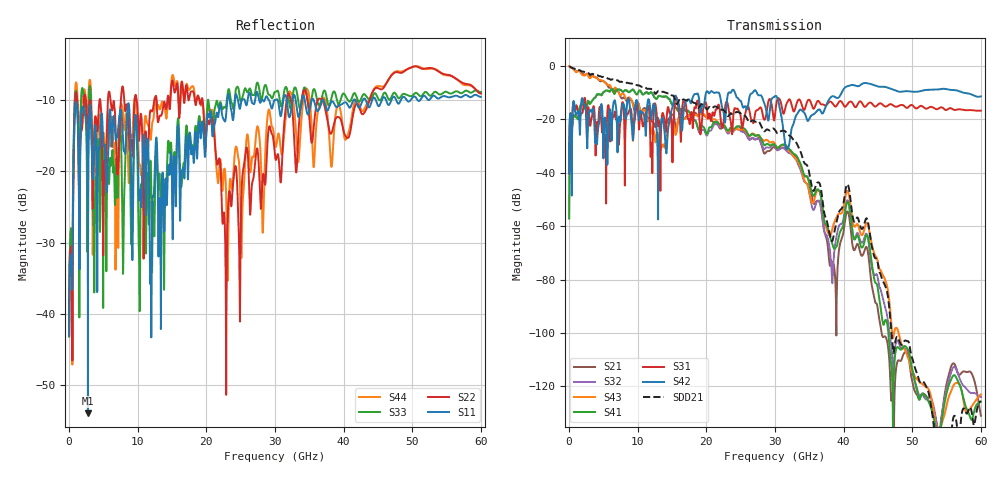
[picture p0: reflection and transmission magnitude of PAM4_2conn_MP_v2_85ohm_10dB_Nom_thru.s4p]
! Info: Touchstone file created by Circ.  Input file=FAB50GbE_2conn_Midplane_Examax_Topo2_v2_85ohm_10dB_Nom.circ
# Hz S RI R 50
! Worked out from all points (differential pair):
!   6000 points, 10 MHz to 60 GHz, reference 50 ohm
!   strongest paths, dB at 10 MHz, 15.01 GHz, 30.01 GHz, 45.01 GHz, 60 GHz:
!     S42: -40.2, -15.9, -11.3, -7.7, -11.4
!     S31: -40.3, -28.2, -18.4, -14.5, -16.7
!     S41: -57.1, -14.4, -29.7, -83.7, -125.7
!     S43: -0.1, -20.4, -29.2, -73.8, -123.0
!     S32: -57.1, -14.5, -30.1, -79.8, -124.0
!     S21: -0.1, -18.2, -30.7, -91.5, -131.0
!   taken as a pair (ports 3,1 in; 4,2 out), SDD21 dB: -0.1, -11.1, -24.0, -74.3, -125.5
!   lowest |S11| = -53.9 dB at 2.75 GHz (marker M1), VSWR 1.00, Z = 50.2 + j0.0695 ohm
!   |S11| at or under -10 dB: start of sweep to 23.06 GHz; 35.65 GHz to 36.88 GHz (1.236 GHz wide, 3.41 % of centre); 37.06 GHz to 41.45 GHz (4.386 GHz wide, 11.2 % of centre)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
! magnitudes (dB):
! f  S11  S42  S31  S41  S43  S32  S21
! 10 MHz  -43.0  -40.2  -40.3  -57.1  -0.1  -57.1  -0.1
! 2.75 GHz  -53.9  -22.9  -16.1  -13.3  -3.4  -13.1  -3.1
! 32.29 GHz  -11.8  -25.4  -13.3  -31.6  -32.3  -32.8  -32.0
! 38.83 GHz  -10.9  -11.8  -15.2  -68.1  -57.4  -65.8  -82.7
! 40.55 GHz  -10.6  -7.6  -14.3  -50.9  -46.8  -50.3  -54.5
! 46.17 GHz  -10.0  -7.9  -15.2  -95.1  -81.0  -91.4  -101.8
! 60 GHz  -9.6  -11.4  -16.7  -125.7  -123.0  -124.0  -131.0
